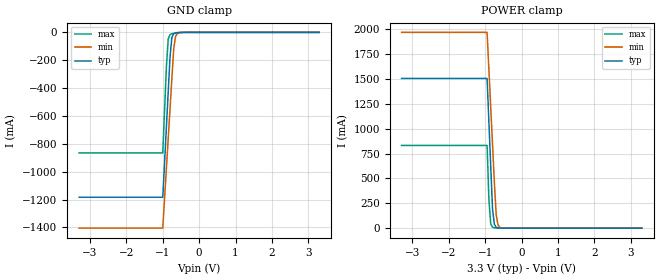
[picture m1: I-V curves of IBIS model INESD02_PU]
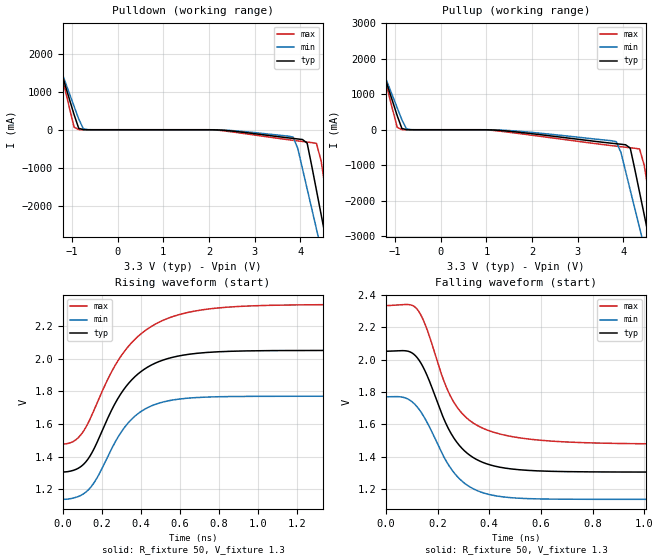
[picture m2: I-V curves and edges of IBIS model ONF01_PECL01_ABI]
|   This file is an IBIS representation of the   |
|   Integrated Devices Technology, Inc.   |
|   ICS843031   |
|   FEMTOCLOCKS CRYSTAL-TO-3.3V LVPECL CLOCK GENERATOR   |
[IBIS Ver]   4.1
[File name]   843031_3v3.ibs
[File Rev]   1.0
[Date]   24 Dec 2008 | Last modified
|   24 Dec 2008 | Generated
[Source]   Originated at Integrated Devices Technology, Inc.
[Disclaimer]
IDT hereby grants the user of this IBIS model a non-exclusive,
nontransferable license to use this IBIS model under the following terms.
Before using this IBIS model, the user should read this license.
If the user does not accept these terms,  the IBIS model should be
returned to IDT within 30 days.
   The user is granted this license only to use the IBIS model and
is not granted rights to sell, load, rent, lease or license the IBIS
model in whole or in part, or in modified form to anyone other than
user. User may modify the IBIS model to suit its specific
applications but rights to derivative works and such modifications
shall belong to IDT.
   This IBIS model is provided on an "AS IS" basis and IDT makes
absolutely no warranty with respect to the information contained
herein. IDT DISCLAIMS AND CUSTOMER WAIVES ALL WARRANTIES, EXPRESS
OR IMPLIED, INCLUDING WARRANTIES OF MERCHANTABILITY OR FITNESS FOR
A PARTICULAR PURPOSE. The entire risk as to quality and performance
is with the Customer. ACCORDINGLY, IN NO EVENT SHALL THE COMPANY BE
LIABLE FOR ANY DAMAGES, WHETHER IN CONTRACT OR TORT,INCLUDING ANY
LOST PROFITS OR OTHER INCIDENTAL, CONSEQUENTIAL, EXEMPLARY, OR
PUNITIVE DAMAGES ARISING OUT OF THE USE OR APPLICATION OF THE IBIS
model provided in this package. Further, IDT reserves the right to
make changes without notice to any product herein to improve
reliability, function, or design. IDT does not convey any license
under patent rights or any other intellectual property rights,
including those of third parties.
   IDT is not obligated to provide maintenance or support
for the licensed IBIS model.
[Copyright]   Copyright 2004 byIntegrated Devices Technology, Inc.
[Component]   ICS843031
[Manufacturer] Integrated Devices Technology, Inc.
[Package]
|TSSOP 8 Lead
|   typ   min   max
R_pkg   52.5m   48.8m   56.2m
L_pkg   1.381nH   1.275nH   1.486nH
C_pkg   0.236pF   0.230pF   0.242pF
[Pin]   signal_name   model_name   R_pin   L_pin   C_pin
1   VCCA   POWER   56.2m   1.486n   0.242p
2   VEE   GND   48.8m   1.275n   0.230p
3   XTAL_OUT   NC   48.8m   1.275n   0.230p
4   XTAL_IN   NC   56.2m   1.468n   0.242p
5   PWR_DN   INESD02_PU   56.2m   1.486n   0.242p
6   nQ0   ONF01_PECL01_ABI   48.8m   1.275n   0.230p
7   Q0   ONF01_PECL01_ABI   48.8m   1.275n   0.230p
8   VCC   POWER   56.2m   1.468n   0.242p
[Diff Pin]  inv_pin  vdiff tdelay_typ tdelay_min  tdelay_max
7   6   NA   0  0  0
| Models and submodels in the file (2): INESD02_PU (Input), ONF01_PECL01_ABI (Output_ECL)
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[Model]   INESD02_PU
Model_type   Input
Polarity   Non-Inverting
Vinl = 0.80V
Vinh = 2.0V
|   typ   min   max
C_comp   2pF   1.5pF   2.5pF
|   typ   min   max
[Voltage range]  3.3V   3.15V   3.45V
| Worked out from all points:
|   GND clamp passes 1 mA (typ) near -0.56 V on its own axis
|   POWER clamp passes 1 mA (typ) near -0.61 V on its own axis
[GND_clamp]
|Voltage   I(typ)   I(min)   I(max)
-3.3V     -1.184A    -1.405A    -865.6mA
-1V       -1.184A    -1.405A    -865.6mA
-900mV    -678.5mA   -975.1mA   -244.1mA
-850mV    -426.2mA   -760.2mA   -46.92mA
-800mV    -174mA     -545.4mA   -16.17mA
-750mV    -37.03mA   -330.8mA   -9.981mA
-700mV    -9.767mA   -120.3mA   -7.122mA
-650mV    -3.616mA   -29.78mA   -4.922mA
-600mV    -1.7mA     -7.594mA   -3.115mA
-400mV    -123.9uA   -126uA     -173.9uA
3.3V      1.866nA    3.949uA    0A
[POWER_clamp]
|Voltage   I(typ)   I(min)   I(max)
-3.3V     1.506A     1.97A      832.1mA
-950mV    1.506A     1.97A      832.1mA
-900mV    1.063A     1.592A     287.2mA
-850mV    620.4mA    1.215A     41.77mA
-800mV    191.5mA    837.4mA    8.692mA
-750mV    37.69mA    460.1mA    3.262mA
-700mV    8.032mA    133.8mA    1.662mA
-650mV    2.005mA    32.58mA    840.1uA
-600mV    607uA      8.009mA    378.6uA
-450mV    33.11uA    139.8uA    23.88uA
3.3V      -71.13uA   -77.46uA   -62.11uA
[Model]   ONF01_PECL01_ABI
Model_type  Output_ECL
Polarity   Non-Inverting
Vmeas = 1.63
Rref = 50
Cref = 0
Vref = 1.3
|Variable  typ   min   max
C_comp   2p   1.5p   2.5p
[Voltage Range]   3.3   3.135   3.465
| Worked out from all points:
|   rising waveform, R_fixture 50, V_fixture 1.3: 20-80 % time 218ps typ, 193ps min, 263ps max; typ from 1.31 V to 2.05 V
|   falling waveform, R_fixture 50, V_fixture 1.3: 20-80 % time 134ps typ, 136ps min, 142ps max; typ from 2.05 V to 1.31 V
| Open source, no load
|  Voltage   I(typ)   I(min)   I(max)
[Pulldown]
-3.3V     9.786A     8.425A     12.06A
-1.667V   3.247A     2.986A     3.704A
-1.463V   2.432A     2.308A     2.661A
-952.6mV  398mA      618.5mA    68.87mA
-850.5mV  36.63mA    281.6mA    4.032mA
3.844V    -229.1mA   -195.7mA   -279.4mA
4.151V    -352.7mA   -1.559A    -324.9mA
4.355V    -1.599A    -2.62A     -360.9mA
4.559V    -2.871A    -3.681A    -1.635A
4.661V    -3.508A    -4.211A    -2.446A
4.763V    -4.144A    -4.742A    -3.257A
6.6V      -15.69A    -14.35A    -17.99A
[Pullup]
-3.3V     9.786A     8.425A     12.06A
-1.565V   2.839A     2.647A     3.182A
-952.6mV  398mA      618.5mA    68.87mA
-850.5mV  36.63mA    281.6mA    4.032mA
-646.4mV  229.3uA    964.8uA    177.5uA
3.844V    -394.4mA   -337mA     -463.1mA
4.151V    -517.8mA   -1.701A    -507.4mA
4.355V    -1.764A    -2.763A    -542.7mA
4.559V    -3.036A    -3.825A    -1.816A
4.661V    -3.672A    -4.355A    -2.626A
4.763V    -4.308A    -4.886A    -3.437A
6.6V      -15.79A    -14.46A    -18.06A
[Ramp]
|   typ   min   max
dV/dt_r   0.596/0.354n   0.506/0.311n   0.684/0.427n
dV/dt_f   0.599/0.219n   0.507/0.219n   0.690/0.252n
R_load =   50.0000
[Rising Waveform]
R_fixture = 50
V_fixture = 1.3   | VCC_typ - 2V
V_fixture_max = 1.465   | VCC_max - 2V
V_fixture_min = 1.135   | VCC_min - 2V
C_fixture = 0.0p
| Time   typ   min   max
0s        1.306V     1.138V     1.478V
67.2ps    1.321V     1.15V      1.503V
126ps     1.379V     1.19V      1.597V
176.4ps   1.489V     1.271V     1.731V
247.8ps   1.679V     1.442V     1.915V
338.1ps   1.85V      1.61V      2.079V
430.5ps   1.946V     1.698V     2.18V
554.4ps   2.007V     1.745V     2.255V
936.6ps   2.049V     1.77V      2.324V
1.999ns   2.052V     1.771V     2.333V
[Falling Waveform]
R_fixture = 50
V_fixture = 1.3   | VCC_typ - 2V
V_fixture_max = 1.465   | VCC_max - 2V
V_fixture_min = 1.135   | VCC_min - 2V
C_fixture = 0.0p
| Time   typ   min   max
0s        2.052V     1.771V     2.334V
73.5ps    2.055V     1.765V     2.34V
119.7ps   2.015V     1.711V     2.314V
151.2ps   1.932V     1.637V     2.221V
224.7ps   1.633V     1.399V     1.868V
268.8ps   1.503V     1.293V     1.723V
336ps     1.398V     1.205V     1.611V
434.7ps   1.338V     1.157V     1.544V
806.4ps   1.307V     1.138V     1.486V
1.999ns   1.306V     1.138V     1.478V
